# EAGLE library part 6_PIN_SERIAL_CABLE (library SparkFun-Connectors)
6-pin header connection for use with the "FTDI BASIC" pinout - CABLE SIDE. Also known as "Arduino Serial Program Header". This is used on a design to provide a 6-pin connection point for serial communication usually from a USB cable (D+/D-) to these headers (RX/TX). It also has the remaining pins necessary for programming in the Arduino evironment (DTR, GND, and sometimes VCC). Note, this device has "CABLE" in the name. It is intended to be used on a design that usually lives on the end of your USB cable and prvides the converter chip (FTDI232 or FTDI231x) to commnicate serial RX/TX. The "sister" device, named "TARGET" is inteneded to be used on a design that contains a target micro-controller that you wish to program. You can populate with some of these: Female Headers (PRT-00115) For reference (or to suit your programming needs) check out these designs: SparkFun FTDI Basic Breakout - 5V (DEV-09716) SparkFun FTDI Basic Breakout - 3.3V (DEV-09873) SparkFun FTDI SmartBasic (DEV-12935) SparkFun Beefy 3 - FTDI Basic Breakout (DEV-13746)
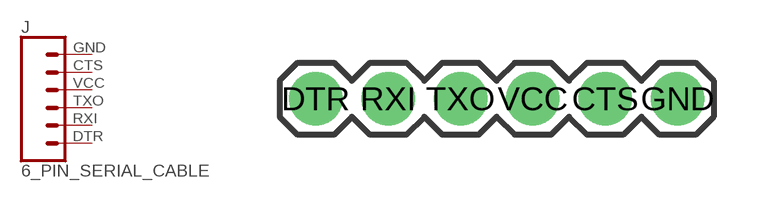
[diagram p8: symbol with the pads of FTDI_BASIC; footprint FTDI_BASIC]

Designator prefix J

## 6_PIN_SERIAL_CABLEPTH  [FTDI_BASIC]
CTS  5  pas
DTR  1  pas
GND  6  pas
RXI  2  pas
TXO  3  pas
VCC  4  pas

## Footprint FTDI_BASIC (pad centres in mm)
FTDI Basic Includes tDocu labels for end pins that match the FTDI Basic connection. Specifications: Pin count: 6 Pin pitch: 0.1" Example device(s): 6_Pin_Serial_Cable
drill 1.016 pad 1.88: CTS 10.16,0; DTR 0,0; GND 12.7,0; RXI 2.54,0; TXO 5.08,0; VCC 7.62,0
